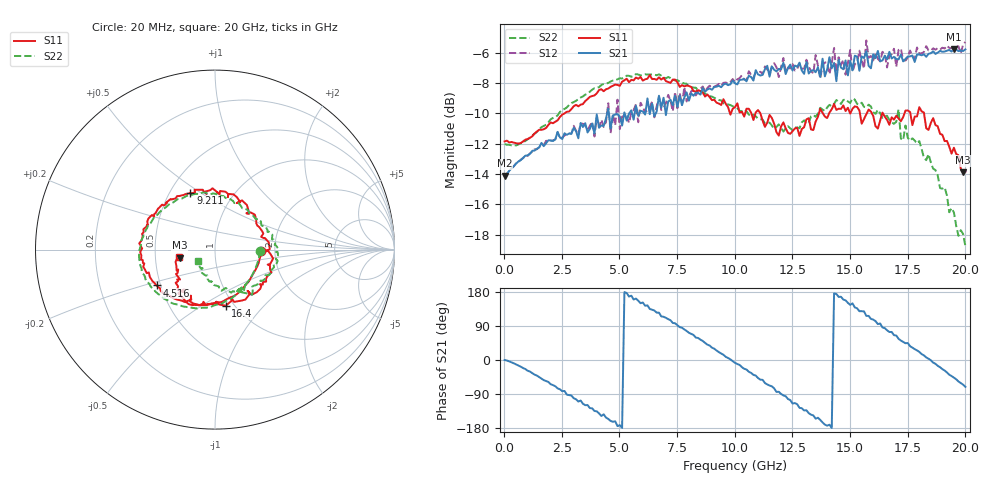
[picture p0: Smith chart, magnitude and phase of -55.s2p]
!Agilent Technologies,N5230A,US43500223,A.07.50.48
!Agilent N5230A: A.07.50.48
!Date: Sunday, September 13, 2015 19:13:21
!Correction: S11(Full 2 Port(1,2))
!S21(Full 2 Port(1,2))
!S12(Full 2 Port(1,2))
!S22(Full 2 Port(1,2))
!S2P File: Measurements: S11, S21, S12, S22:
# Hz S  dB  R 50
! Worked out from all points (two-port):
!   201 points, 20 MHz to 20 GHz, reference 50 ohm
!   highest |S21| = -5.74 dB at 19.5 GHz (marker M1); lowest = -14.1 dB at 20 MHz (marker M2)
!   |S21| within 3 dB of the highest: 8.254 GHz to 8.499 GHz (245.3 MHz wide, 2.93 % of centre); 8.515 GHz to end of sweep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
!   lowest |S11| = -13.9 dB at 19.9 GHz (marker M3), VSWR 1.51, Z = 33.4 - j3.19 ohm
!   |S11| at or under -10 dB: start of sweep to 2.609 GHz; 11.11 GHz to 13.65 GHz (2.536 GHz wide, 20.5 % of centre); 18.21 GHz to end of sweep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
!   |S22| runs from -18.8 to -7.4 dB; largest |S21 - S12| = 0.092
!   S11 on the Smith chart (normalised r, x): 20 MHz: 1.69, -0.02; 4.516 GHz: 0.48, -0.22; 9.211 GHz: 0.63, +0.45; 16.4 GHz: 0.92, -0.64; 20 GHz: 0.67, -0.06
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2e7  -11.85 -1.5  -14.11 0.0  -14.15 -0.1  -12.02 -1.7
1.5185e9  -11.08 -66.9  -12.24 -45.1  -12.23 -45.3  -11.07 -67.0
3.4166e9  -9.38 -123.2  -10.90 -115.5  -10.68 -118.7  -8.87 -118.0
4.5155e9  -8.36 -148.5  -9.68 -155.6  -9.32 -155.1  -7.98 -140.7
4.6154e9  -8.24 -152.4  -10.99 -160.8  -11.31 -161.7  -7.89 -142.9
4.9151e9  -8.12 -157.9  -10.05 -174.5  -9.09 -175.6  -7.75 -148.3
5.015e9  -8.18 -161.0  -10.20 -172.0  -11.03 -173.5  -7.68 -150.0
6.7133e9  -7.62 167.9  -8.83 124.9  -8.89 124.6  -7.42 -178.1
7.8122e9  -8.22 148.5  -8.95 80.6  -8.26 79.0  -8.03 162.4
9.2108e9  -9.29 113.5  -8.24 25.0  -8.15 23.8  -9.06 132.7
1.001e10  -9.58 94.6  -8.01 -7.5  -7.93 -8.3  -9.58 113.2
1.09091e10  -9.93 76.5  -7.14 -41.1  -7.29 -42.0  -10.19 88.4
1.21079e10  -10.59 41.1  -6.65 -93.5  -6.34 -95.1  -11.19 56.6
1.34066e10  -11.10 -0.2  -7.14 -146.3  -7.37 -144.2  -10.11 20.5
1.43057e10  -9.38 -22.0  -6.66 175.9  -5.67 176.8  -9.37 4.0
1.56044e10  -10.37 -51.4  -6.35 128.3  -7.03 122.0  -9.57 -20.6
1.64036e10  -9.94 -79.2  -6.50 85.9  -5.93 86.6  -10.28 -34.5
1.67033e10  -10.75 -88.5  -5.93 73.9  -6.17 75.8  -10.42 -41.4
1.83017e10  -10.98 -128.2  -6.26 6.7  -5.56 3.3  -13.08 -74.7
1.95005e10  -12.26 -151.2  -5.74 -46.5  -5.59 -50.2  -16.53 -119.0
1.99001e10  -13.87 -166.9  -5.88 -65.0  -5.44 -68.7  -17.95 -139.9
2e10  -13.84 -167.6  -5.77 -70.9  -5.28 -74.4  -18.76 -147.6
